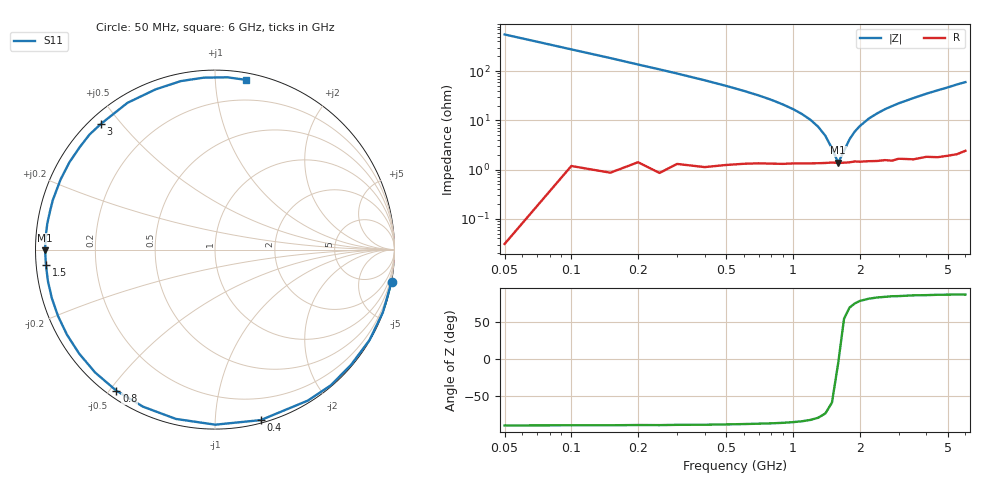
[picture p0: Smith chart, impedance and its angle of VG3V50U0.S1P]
! Infineon Technologies  Discrete & RF Semiconductors
! BB 831
! Si Tuning Diode in SOD323
! VR = 3.5 V
! S-Parameters:  July  1999
# GHz  S  MA  R  50
!  f  S11
! GHz  MAG  ANG
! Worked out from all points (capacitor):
!   34 points, 50 MHz to 6 GHz, reference 50 ohm
!   read as one part to ground: C = 5.73 pF near 50 MHz
!   lowest |Z| = 1.37 ohm at 1.6 GHz (marker M1)
!   series resonance near 1.606 GHz, so ESL is about 1.7 nH
!   S11 on the Smith chart (normalised r, x): 50 MHz: 0, -11; 400 MHz: 0.02, -1.30; 800 MHz: 0.03, -0.52; 1.5 GHz: 0.03, -0.05; 3 GHz: 0.03, +0.44; 6 GHz: 0.05, +1.19
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0.05  1 -10.3
0.1  0.9985 -20.5
0.15  0.9976 -30.4
0.2  0.9933 -40.3
0.25  0.994 -49.5
0.3  0.9877 -58.4
0.4  0.9835 -75.0
0.5  0.9755 -89.9
0.6  0.9683 -103.0
0.7  0.9626 -114.6
0.8  0.9592 -124.9
0.9  0.9565 -134.3
1  0.9532 -142.6
1.1  0.9514 -150.1
1.3  0.9485 -163.4
1.5  0.9458 -174.7
1.6  0.9467 -179.7
1.8  0.9456 171.1
2  0.9449 163.0
2.4  0.9458 149.1
2.6  0.9454 142.9
3  0.9458 132.2
3.5  0.9522 120.8
4  0.952 110.4
4.5  0.958 101.5
5  0.9599 93.8
5.5  0.9625 85.9
6  0.9611 79.8
